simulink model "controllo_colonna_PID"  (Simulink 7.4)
settings: Solver=ode45  StartTime=0.0  StopTime=100.0  RelTol=1e-4
libraries: cstblocks x2

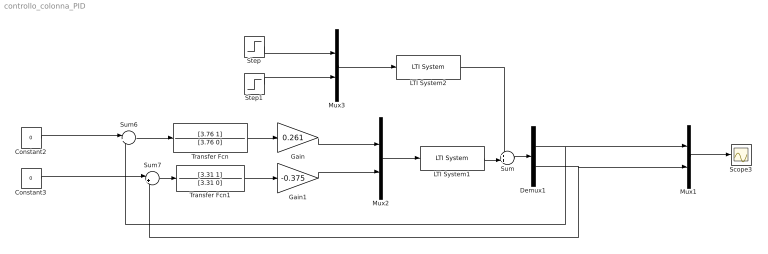
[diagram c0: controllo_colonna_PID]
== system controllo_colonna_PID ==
  Constant2 : Constant  Value=0  OutDataType=sfix(16)  OutScaling=2^0
  Constant3 : Constant  Value=0  OutDataType=sfix(16)  OutScaling=2^0
  Demux1 : Demux  Outputs=2
  Gain : Gain  Gain=0.261  ParameterDataType=fixdt(1, 16)  ParameterScaling=2^0  OutDataType=fixdt(1, 16)  OutScaling=2^0
  Gain1 : Gain  Gain=-0.375  ParameterDataType=fixdt(1, 16)  ParameterScaling=2^0  OutDataType=fixdt(1, 16)  OutScaling=2^0
  LTI System1 : cstblocks/LTI System  SystemSampleTime=-1  sys=G  IC=[]
  LTI System2 : cstblocks/LTI System  SystemSampleTime=-1  sys=Gd  IC=[]
  Mux1 : Mux  Inputs=2
  Mux2 : Mux  Inputs=2
  Mux3 : Mux  Inputs=2
  Scope3 : Scope
  Step : Step  Time=0  After=2/3  SampleTime=0
  Step1 : Step  Time=50  After=1/2  SampleTime=0
  Sum : Sum  Inputs=++|  OutDataType=fixdt(1, 16)  OutScaling=2^0
  Sum6 : Sum  Inputs=|+-  OutDataType=sfix(16)  OutScaling=2^0
  Sum7 : Sum  Inputs=|+-  OutDataType=sfix(16)  OutScaling=2^0
  Transfer Fcn : TransferFcn  Numerator=[3.76 1]  Denominator=[3.76 0]
  Transfer Fcn1 : TransferFcn  Numerator=[3.31 1]  Denominator=[3.31 0]
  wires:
  Mux2/1 -> LTI System1/1
  Mux1/1 -> Scope3/1
  Demux1/1 -> Mux1/1, Sum6/2
  Sum6/1 -> Transfer Fcn/1
  Sum7/1 -> Transfer Fcn1/1
  Demux1/2 -> Mux1/2, Sum7/2
  Constant2/1 -> Sum6/1
  Constant3/1 -> Sum7/1
  Gain/1 -> Mux2/1
  Transfer Fcn/1 -> Gain/1
  Transfer Fcn1/1 -> Gain1/1
  Gain1/1 -> Mux2/2
  Sum/1 -> Demux1/1
  LTI System1/1 -> Sum/2
  LTI System2/1 -> Sum/1
  Mux3/1 -> LTI System2/1
  Step/1 -> Mux3/1
  Step1/1 -> Mux3/2
